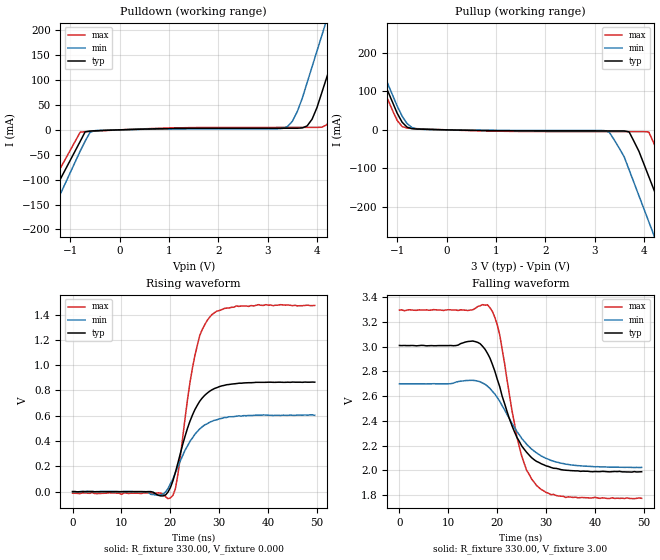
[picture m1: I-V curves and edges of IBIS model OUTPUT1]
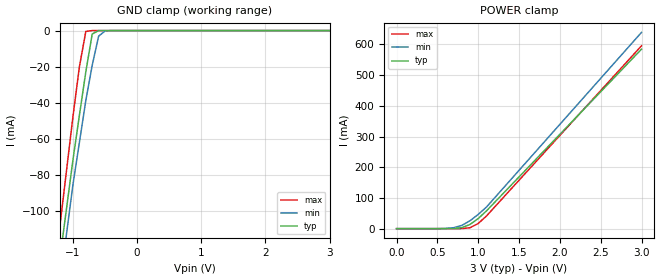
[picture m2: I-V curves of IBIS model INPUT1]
| IBIS file 8581nb3v.ibs
[IBIS ver]   2.1
[File name]   8581nb3v.ibs
[File Rev]   1.0
[Date]   July 4, 2003
[Source]   This file orginated at SEIKO EPSON QD Div.
   This file is for 3.0V CMOS parts.
[Copyright]   Copyright SEIKO EPSON Corp. 2003
|   Component RX-8581NB
[Component]   RX-8581NB
[Manufacturer]   SEIKO EPSON
[Package]
| variable   typ   min   max
R_pkg   87m   NA   NA
L_pkg   10nH   NA   NA
C_pkg   206fF   NA   NA
[Pin]  signal_name   model_name   R_pin   L_pin   C_pin
|1   /INT
2   GND   GND
|3   (VDD)
|4   NC
|5   SDA
|6   SCL
7   FOUT   OUTPUT1
8   VDD   POWER
9   FOE   INPUT1
| Models and submodels in the file (2): OUTPUT1 (Output), INPUT1 (Input)
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|10   NC
|11   NC
|12   NC
|13   NC
|14   NC
|15   NC
|16   NC
|17   NC
|18   NC
|19   NC
|20   NC
|21   NC
|22   NC
|   Model OUTPUT
[Model]   OUTPUT1
Model_type   Output
Polarity   Non-Inverting
Enable   Active-High
Vmeas =   1.50V
C_comp   1.69pF   1.32pF   1.96pF
[Temperature Range]   25.00   85.00   -40.000
[Voltage Range]   3.0V   2.7V   3.3V
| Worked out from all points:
|   slope of the pulldown table from 0 to 0.45 V, typ, clamps not added: 333 ohm
|   slope of the pullup table from 0 to 0.45 V, typ, clamps not added: 391 ohm
|   rising waveform, R_fixture 330.00, V_fixture 0.000: 20-80 % time 4.48ns typ, 4.95ns min, 3.57ns max; typ from 0 V to 0.865 V
|   falling waveform, R_fixture 330.00, V_fixture 3.00: 20-80 % time 5.61ns typ, 7.03ns min, 4.37ns max; typ from 3.01 V to 1.99 V
[Pulldown]
| voltage   I(typ)   I(min)   I(max)
-3V       -437.3mA   -514.5mA   -401mA
-1.9V     -230.2mA   -278.6mA   -202.9mA
-1.6V     -173.8mA   -214.2mA   -148.8mA
-800mV    -23.2mA    -42.7mA    -4.7mA
-500mV    -1.9mA     -1.6mA     -2.5mA
3.4V      3.2mA      6.6mA      4.9mA
3.8V      7.9mA      94.8mA     4.9mA
4.1V      75.5mA     190.2mA    5.3mA
4.3V      136.7mA    253.9mA    27.6mA
4.5V      197.9mA    317.5mA    89.1mA
4.9V      320.3mA    444.7mA    221.3mA
6V        657mA      794.7mA    585mA
[Pullup]
| voltage   I(typ)   I(min)   I(max)
-3V       650.8mA    670.7mA    625.6mA
-1.9V     316.6mA    335.9mA    293.6mA
-1.7V     255.9mA    275mA      233.2mA
-1V       43.2mA     62mA       24.5mA
-800mV    7mA        16.4mA     4.5mA
3.3V      -2.8mA     -6.5mA     -4.7mA
3.7V      -5.3mA     -104mA     -4.7mA
4.1V      -122mA     -239.6mA   -5.6mA
4.2V      -155mA     -273.5mA   -34.4mA
4.5V      -254mA     -375.2mA   -121.7mA
5V        -419mA     -544.7mA   -267.2mA
6V        -749mA     -883.7mA   -558.2mA
[Ramp]
| variable   typ   min   max
dV/dt_r 0.52/4.5n   0.36/5n 0.89/3.4n
dV/dt_f 0.61/5.6n   0.41/7n 0.91/4.4n
R_load = 330.00
[Rising Waveform]
R_fixture = 330.00
V_fixture = 0.000
| time   V(typ)   V(min)   V(max)
0s        0V         0V         -12mV
17.5ns    -28mV      -30mV      -10mV
20ns      32mV       63mV       -50mV
21.5ns    222mV      192mV      128mV
23.5ns    502mV      361mV      730mV
25ns      648mV      453mV      1.076V
26ns      715mV      496mV      1.236V
27.5ns    778mV      536mV      1.353V
33.5ns    854mV      596mV      1.468V
49.5ns    865mV      603mV      1.472V
[Falling Waveform]
R_fixture = 330.00
V_fixture = 3.00
V_fixture_min = 2.70
V_fixture_max = 3.30
| time   V(typ)   V(min)   V(max)
0s        3.01V      2.7V       3.296V
15ns      3.046V     2.728V     3.299V
18ns      2.946V     2.681V     3.339V
19.5ns    2.802V     2.617V     3.237V
20.5ns    2.676V     2.559V     3.095V
23ns      2.361V     2.379V     2.483V
25ns      2.197V     2.258V     2.115V
28ns      2.073V     2.142V     1.879V
34ns      2.001V     2.05V      1.781V
49.5ns    1.989V     2.024V     1.774V
|   Model INPUT1
[Model]   INPUT1
Model_type   Input
Polarity   Non-Inverting
Vinl =   1.00V
Vinh =   2.20V
C_comp   0.80pF   0.60pF   1.00pF
[Temperature Range]   25.00   85.00   -40.00
[Voltage Range]   3.00V   2.70V   3.30V
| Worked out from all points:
|   GND clamp passes 1 mA (typ) near -0.65 V on its own axis
[GND_clamp]
| voltage   I(typ)   I(min)   I(max)
-3V       -609.6mA   -631.3mA   -643.6mA
-1.3V     -152.3mA   -167.2mA   -137mA
-1.2V     -125.4mA   -139.9mA   -107.2mA
-1.1V     -98.5mA    -112.6mA   -77.4mA
-1V       -71.6mA    -85.3mA    -47.6mA
-900mV    -47mA      -62.1mA    -20.1mA
-800mV    -22.9mA    -38.8mA    -500uA
-700mV    -1.9mA     -19.2mA    0A
-600mV    0A         -3.1mA     0A
-500mV    0A         -200uA     0A
3V        0A         0A         0A
[POWER_clamp]
| voltage   I(typ)   I(min)   I(max)
0V        0A         0A         0A
500mV     0A         100uA      0A
700mV     500uA      3.1mA      0A
800mV     3.3mA      10.7mA     200uA
900mV     13.7mA     25.8mA     3.1mA
1V        32.9mA     46.4mA     16.8mA
1.1V      57.5mA     70.1mA     40.9mA
3V        584.5mA    639.1mA    595.5mA
